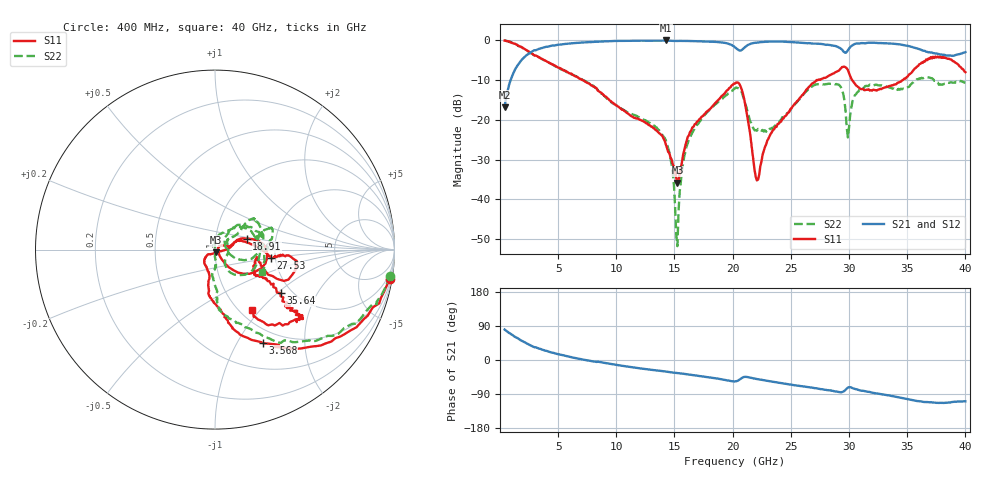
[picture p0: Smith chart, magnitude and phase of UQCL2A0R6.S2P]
! AVX Corporation
! Date:  10/27/06
! Part No:  UQCL2A0R6
! Description:  Ultra Low ESR Microwave capacitors
! Mounting Orientation:  Horizontal
# GHZ S DB R 50
! Freq  |S11|  S11 Ph  |S21|  S21 Ph  |S12|  S12 Ph  |S22|  S22 Ph
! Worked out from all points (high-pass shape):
!   401 points, 400 MHz to 40 GHz, reference 50 ohm
!   highest |S21| = -0.11 dB at 14.26 GHz (marker M1); lowest = -16.8 dB at 400 MHz (marker M2)
!   |S21| within 3 dB of the highest: 2.632 GHz to 29.64 GHz (27.01 GHz wide, 167 % of centre); 29.75 GHz to 36.99 GHz (7.239 GHz wide, 21.7 % of centre)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
!   lowest |S11| = -35.8 dB at 15.25 GHz (marker M3), VSWR 1.03, Z = 50.3 - j1.59 ohm
!   |S11| at or under -10 dB: 7.033 GHz to 27.36 GHz (20.33 GHz wide, 118 % of centre); 30.26 GHz to 34.64 GHz (4.383 GHz wide, 13.5 % of centre)
!   |S22| runs from -51.8 to -0.1 dB; largest |S21 - S12| = 0.013
!   S11 on the Smith chart (normalised r, x): 400 MHz: 1, -12; 3.568 GHz: 0.81, -1.29; 18.91 GHz: 1.42, +0.18; 27.53 GHz: 1.90, -0.20; 35.64 GHz: 1.74, -1.05; 40 GHz: 1.13, -0.90
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0.4  -0.11 -9.4  -16.84 80.3  -16.85 80.3  -0.10 -8.6
1.588  -1.41 -34.7  -6.05 56.2  -6.10 55.5  -1.50 -31.4
3.568  -4.67 -62.9  -2.04 28.3  -2.02 27.9  -4.71 -58.5
7.033  -10.00 -87.5  -0.64 1.8  -0.60 2.1  -9.80 -86.4
13.666  -23.36 -140.2  -0.18 -28.3  -0.17 -28.4  -22.60 -88.2
14.26  -26.27 -145.9  -0.11 -30.6  -0.12 -30.4  -25.25 -86.5
15.25  -35.81 -77.2  -0.23 -34.2  -0.23 -34.0  -51.76 64.9
16.24  -23.89 0.4  -0.24 -38.4  -0.23 -38.3  -24.98 89.0
18.913  -14.59 19.0  -0.54 -50.2  -0.56 -50.0  -15.18 45.9
20.2  -10.92 -1.2  -1.82 -56.5  -1.79 -56.3  -12.13 7.1
20.893  -13.59 -40.1  -2.22 -45.5  -2.25 -45.4  -14.13 -46.3
22.081  -35.24 -0.6  -0.65 -50.4  -0.65 -50.2  -22.77 -22.2
23.269  -23.54 16.5  -0.37 -56.5  -0.37 -56.4  -22.34 27.0
26.833  -10.91 -3.1  -0.89 -73.0  -0.81 -72.9  -11.67 39.9
27.526  -9.99 -8.6  -0.96 -76.7  -1.02 -76.8  -11.02 36.9
29.209  -7.42 -5.5  -1.98 -84.9  -1.99 -84.5  -11.46 5.0
29.902  -7.50 -24.4  -2.57 -72.8  -2.59 -72.5  -24.45 19.9
30.892  -12.12 -13.7  -0.83 -79.8  -0.81 -79.5  -12.51 32.1
33.466  -11.51 -31.5  -0.88 -93.6  -0.88 -93.4  -11.92 16.9
35.644  -7.15 -33.8  -1.94 -107.0  -1.90 -106.8  -10.30 21.5
37.822  -4.11 -38.5  -3.61 -113.0  -3.55 -112.7  -11.12 -3.9
40  -8.07 -58.9  -3.03 -109.1  -3.03 -108.9  -10.71 -25.0
